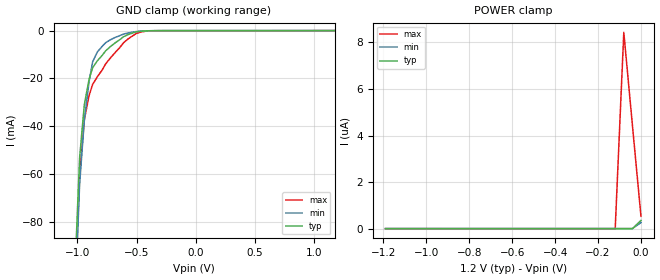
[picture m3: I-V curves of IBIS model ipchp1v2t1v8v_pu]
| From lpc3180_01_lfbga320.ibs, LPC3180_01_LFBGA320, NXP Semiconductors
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| |   Rev 0.20 IBIS Model Design Automation Generation   |
| |   N O N - S I L I C O N   C O R R E L A T E D   |
| |   This IBIS [Model] is pre-Beta tactical support   |
| |  Note: this IBIS [Model] contains clamp curves generated   |
| |   through simulation which should not be relied upon   |
| ipchp1v2t1v8v
|   Input Pad 1v2
|   Push Pull
|   CMOS
|   Programmable between
|   - (p1=0, p2=1) plain input
|   - (p1=0, p2=0) with Pull Up
|   - (p1=1, p2=1) with Pull Down
|   - (p1=1, p2=0) with Repeater
|   Characterized at Core 1.2V and I/O 1.8V
| Pull Up Mode (p1=0, p2=0)
[Model]   ipchp1v2t1v8v_pu | of ipchp1v2t1v8v
Model_type   Input
|  Reciever Thresholds
Vinl   = 0.36V
Vinh   = 0.84V
| [Process Range]   typical   min   max
| C_comp edge width   400.000ps   400.000ps   400.000ps
| C_comp Tstrobe   40.000fs   40.000fs   40.000fs
C_comp   2.020pF   1.887pF   2.187pF
[Temperature Range]   25   105   -20
[Voltage Range]   1.20V   1.10V   1.30V
[GND Clamp Reference]   0.00V   0.00V   0.00V
[Pulldown Reference]   0.00V   0.00V   0.00V
[POWER Clamp Reference]   1.20V   1.10V   1.30V
[Pullup Reference]   1.20V   1.10V   1.30V
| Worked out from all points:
|   GND clamp passes 1 mA (typ) near -0.53 V on its own axis
[GND Clamp]
| ref voltage   0.00V   0.00V   0.00V
|   Voltage   I(typ)   I(min)   I(max)
-1.2V     -373.8mA   -377.3mA   -396.4mA
-1.01V    -89.19mA   -101.8mA   -99.48mA
-980mV    -53.06mA   -64.23mA   -60.46mA
-940mV    -30.85mA   -37.28mA   -37.23mA
-900mV    -20.29mA   -21.21mA   -27.11mA
-870mV    -15.47mA   -13mA      -22.45mA
-830mV    -12.6mA    -8.911mA   -19.26mA
-760mV    -8.427mA   -5.039mA   -13.87mA
-570mV    -1.651mA   -984.3uA   -3.435mA
-500mV    -504.7uA   -388uA     -1.157mA
-420mV    -130.9uA   -135.7uA   -249.3uA
1.17V     -2.217uA   4.528nA    -12.6uA
[Power Clamp]   | Vtable = Vcc - Vpad
| ref voltage   1.20V   1.10V   1.30V
|   Voltage   I(typ)   I(min)   I(max)
-1.19V    523.6pA    5.399nA    478.3pA
-120mV    332.3pA    4.574nA    207pA
-80mV     327.9pA    4.541nA    8.428uA
-40mV     323.1pA    4.489nA    4.455uA
0V        354.1nA    261.6nA    531.4nA
